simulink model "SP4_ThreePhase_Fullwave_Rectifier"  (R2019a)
settings: Solver=VariableStepAuto  StartTime=0  StopTime=0.3  FixedStep=1e-5  RelTol=1e-5
libraries: fl_lib x10, nesl_utility x5, powerlib_meascontrol x1

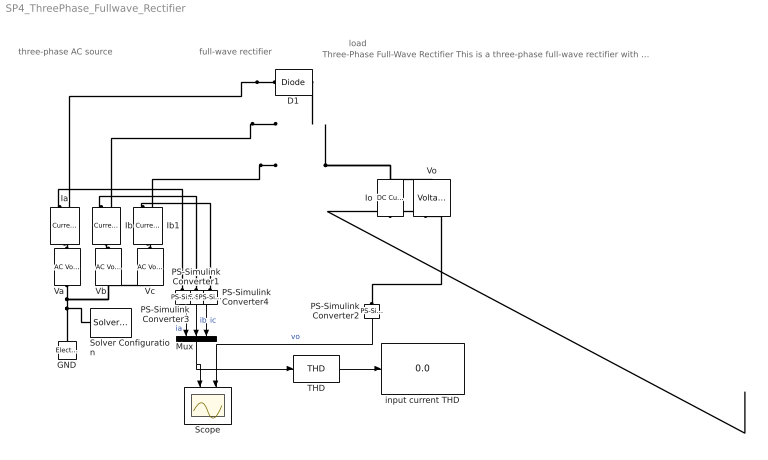
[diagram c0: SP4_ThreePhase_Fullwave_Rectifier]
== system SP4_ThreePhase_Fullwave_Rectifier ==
  note: Three-Phase Full-Wave Rectifier This is a three-phase full-wave rectifier with a constant-current load. 1. One ideal diode is placed, but the other five need to be added. Copy and paste the existing diode. 2. Place the other diodes to make the full-wave rectifier. Press Ctrl+R to rotate a component. C1. Capture the complete circuit diagram. 3. Simulate the circuit (click the Run button above). 4. Open the Scope below (double click). Press the "Scale X & Y Axis Limits" to fit data to the screen. 5. Observe the current and voltage waveforms. C2. Capture the three current (top plot) and one voltage (bottom plot) waveforms. Q1. What is the average output voltage? Q2. What is the output power? 6. The THD block calculates the THD values of the three input currents.. 7. The display shows the input current THD values at the end of the simulation. Q3. What is the THD of each phase of the input current? ------------------------------------------------------- Let's see how the input current is affected by increasing the load current. 8. Double click on output current source (Io) to see it's properties. 9. Increase the constant current value to 10 A. 10. Simulate the circuit again (click the Run button above). 11. Open the Scope (double click). Press the "Scale X & Y Axis Limits" to fit data to the screen. C3. Capture the new current and voltage waveforms. Q4. What is the new output power? Q5. What is the new THD of each phase of the input current? Q6. How does amplitude affect the THD of the input current waveform? Explain briefly. _________________________________ Play: Try changing the load to a resistor or a resistor in parallel with a capacitor. Observe how the shape of the current and voltage waveforms change.
  note: load
  note: three-phase AC source
  note: full-wave rectifier
  D1 : fl_lib/Electrical/Electrical Elements/Diode  Vf=1e-3 V  Ron=1e-3 Ohm  Goff=1e-8 1/Ohm  i_specify=off  i_priority=None  i=0 A  i_nominal_specify=off  i_nominal_unit=A  i_nominal_value=1  v_specify=off  v_priority=None  v=0 V  v_nominal_specify=off  v_nominal_unit=V  v_nominal_value=1
  GND : fl_lib/Electrical/Electrical Elements/Electrical Reference
  Ia : fl_lib/Electrical/Electrical Sensors/Current Sensor
  Ib : fl_lib/Electrical/Electrical Sensors/Current Sensor
  Ib1 : fl_lib/Electrical/Electrical Sensors/Current Sensor
  Io : fl_lib/Electrical/Electrical Sources/DC Current Source  i0=1 A
  Mux : Mux  Inputs=3
  PS-Simulink Converter{1..4} (4 alike) : nesl_utility/PS-Simulink Converter  PhysicalDomain=network_engine_domain  SubClassName=ps_output  LeftPortType=input  RightPortType=output  PseudoPeriodic=off  Frequencies=[]  Unit=1  AffineConversion=off
  Scope : Scope  NumInputPorts=2
  Solver Configuration : nesl_utility/Solver Configuration  PhysicalDomain=network_engine_domain  SubClassName=solver  LeftPortType=input  RightPortType=generic  Tones=[]  Harmonics=[]  SimulateNoise=off  Profile=off  UseLocalSampling=off  EnableSwitchedLinearOptims=on  FrequencyDomain=off  UseCCode=off  RelTol=0.001  AbsTol=1e-06  MinStep=1e-09  ToWorkspace=off  RevertToSquareIcSolve=off  NumHomotopyIterations=100  PhasorMode=off  PhasorModeNumHarmonics=1  DoDC=off  ResidualTolerance=1e-09  UseLocalSolver=off  LocalSolverChoice=NE_BACKWARD_EULER_ADVANCER  LocalSolverSampleTime=0.001  DoFixedCost=off  MaxNonlinIter=3  MaxModeIter=2  LinearAlgebra=auto  EquationFormulation=NE_TIME_EF  DelaysMemoryBudget=1024  AutomaticFiltering=on  FilteringTimeConstant=0.001  PartitionStorageMethod=AS_NEEDED  PartitionMemoryBudget=1024  PartitionMethod=ROBUST
  THD : powerlib_meascontrol/Measurements/THD  Freq=5  Ts=0
  Va : fl_lib/Electrical/Electrical Sources/AC Voltage Source  amp=17 V  shift=0 deg  frequency=5 Hz  omega=0 rad/s
  Vb : fl_lib/Electrical/Electrical Sources/AC Voltage Source  amp=17 V  shift=120 deg  frequency=5 Hz  omega=0 rad/s
  Vc : fl_lib/Electrical/Electrical Sources/AC Voltage Source  amp=17 V  shift=240 deg  frequency=5 Hz  omega=0 rad/s
  Vo : fl_lib/Electrical/Electrical Sensors/Voltage Sensor
  input current THD : Display
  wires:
  Mux/1 -> Scope/1, THD/1
  PS-Simulink Converter4/1 -> Mux/3  "ic"
  PS-Simulink Converter1/1 -> Mux/2  "ib"
  PS-Simulink Converter3/1 -> Mux/1  "ia"
  PS-Simulink Converter2/1 -> Scope/2  "vo"
  THD/1 -> input current THD/1
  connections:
  Va/RConn1 -- Vc/RConn1 -- Vb/RConn1 -- GND/LConn1 -- Solver Configuration/RConn1
  PS-Simulink Converter2/LConn1 -- Vo/RConn1
  D1/RConn1 -- Vo/LConn1 -- Io/RConn1
  D1/LConn1 -- Ia/RConn2
  Ib/RConn2 -- ?
  Ib1/RConn2 -- ?
  Va/LConn1 -- Ia/LConn1
  Ib/LConn1 -- Vb/LConn1
  Vc/LConn1 -- Ib1/LConn1
  Io/LConn1 -- Vo/RConn2
  PS-Simulink Converter3/LConn1 -- Ia/RConn1
  PS-Simulink Converter1/LConn1 -- Ib/RConn1
  PS-Simulink Converter4/LConn1 -- Ib1/RConn1
